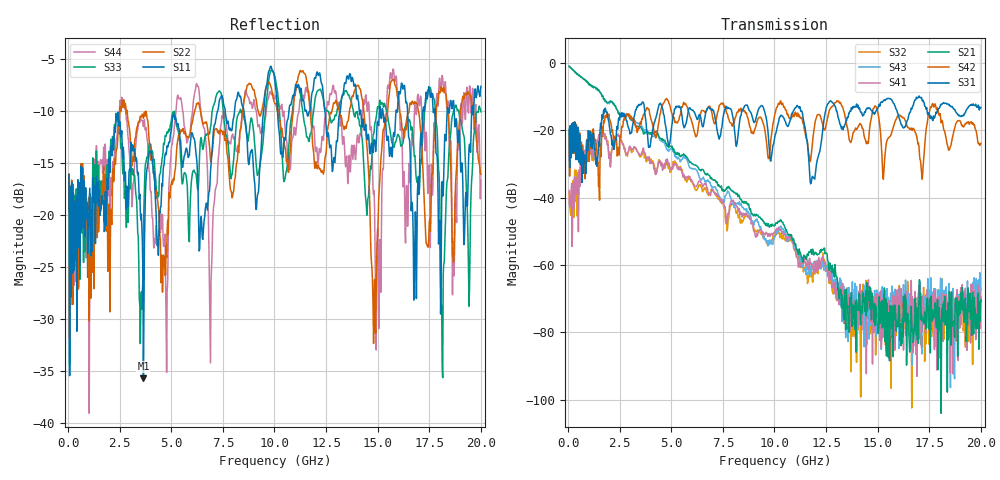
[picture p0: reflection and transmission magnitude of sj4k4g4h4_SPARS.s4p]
! FILE: E:\users\goganessyan\GBX_Backplane\FR408_backplane\1m_OUTBOUND_TRU\sj4k4g4h4_SPARS.s4p
# MHZ S RI R 50.00
! FREQ  S11  S12  S13  S14
!  S21  S22  S23  S24
!  S31  S32  S33  S34
!  S41  S42  S43  S44
!  REAL  IMAG  REAL  IMAG  REAL  IMAG  REAL  IMAG
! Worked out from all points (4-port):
!   799 points, 50 MHz to 20 GHz, reference 50 ohm
!   strongest paths, dB at 50 MHz, 5.025 GHz, 10.03 GHz, 15.03 GHz, 20 GHz:
!     S31: -19.8, -18.6, -21.6, -13.3, -13.4
!     S42: -20.0, -15.0, -15.1, -15.3, -23.9
!     S21: -1.0, -24.7, -48.3, -80.3, -70.3
!     S41: -37.9, -31.0, -50.3, -73.0, -69.4
!     S43: -1.1, -25.5, -51.7, -69.3, -70.1
!     S32: -38.7, -31.3, -51.1, -71.4, -67.3
!   lowest |S11| = -35.7 dB at 3.65 GHz (marker M1), VSWR 1.03, Z = 50 + j1.64 ohm
!   |S11| at or under -10 dB: start of sweep to 7.244 GHz; 8.518 GHz to 9.471 GHz (952.8 MHz wide, 10.6 % of centre); 14.18 GHz to 15.09 GHz (908.2 MHz wide, 6.21 % of centre)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
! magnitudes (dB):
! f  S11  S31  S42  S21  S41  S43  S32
! 50 MHz  -16.1  -19.8  -20.0  -1.0  -37.9  -1.1  -38.7
! 3.65 GHz  -35.7  -11.9  -15.4  -21.0  -25.3  -19.9  -26.1
! 11.15 GHz  -7.4  -13.0  -15.8  -56.4  -60.5  -57.1  -57.6
! 11.8 GHz  -8.5  -34.6  -26.3  -56.8  -59.9  -59.4  -62.2
! 14.43 GHz  -11.3  -14.1  -23.2  -67.7  -74.0  -74.0  -64.5
! 14.85 GHz  -12.8  -15.3  -13.0  -71.5  -74.2  -67.5  -77.2
! 20 GHz  -7.6  -13.4  -23.9  -70.3  -69.4  -70.1  -67.3
